(* Logix 5000 DataType export RTA_435NBX_490NBX; software revision 20.04 *)

TYPE RTA_435NBX_490NBX :
STRUCT
   PLC_to_Gateway : RTA_STRING_4096;   // Controller Scope Tag that the RTA_435NBX_490NBX_PLC_to_Gateway AOI uses to move the raw ASCII message from the ASCII device to the PLC
   Gateway_to_PLC : RTA_STRING_4096;   // Controller Scope Tag that the RTA_435NBX_490NBX_Gateway_to_PLC AOI uses to move the raw ASCII message from the PLC to the ASCII device
   Data_to_Customer : RTA_STRING_4096;   // Contoller Scope Tag that the RTA_435NBX_490NBX_Gateway_to_PLC AOI uses to move the data to for the Customer to process.
   Data_from_Customer : RTA_STRING_4096;   // Contoller Scope Tag that the RTA_435NBX_490NBX_PLC_to_Gateway AOI uses to move the Customer's data in the PLC to the Tag the Gateway is monitoring.
   Active : INT;   // Contoller Scope Tag that the RTA_435NBX_490NBX_Heartbeat AOI uses to let the PLC know that the 435NBX / 490NBX is present and actively communicating to the PLC.
   Heartbeat : INT;   // Contoller Scope Tag that the 435NBX / 490NBX updates to let the PLC know the 435NBX / 490NBX is present and actively communicating.
END_STRUCT
END_TYPE

TYPE RTA_STRING_4096 :   // string type; String Data Type with up to 4096 characters available
STRUCT
   LEN : DINT;
   DATA : SINT[4096];
END_STRUCT
END_TYPE
